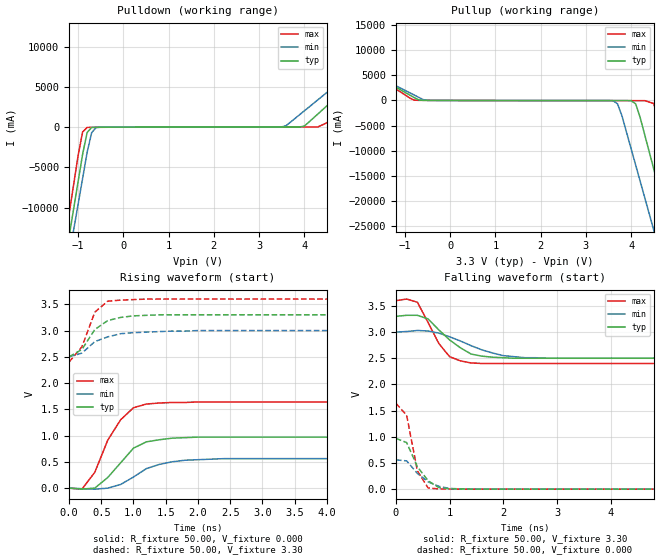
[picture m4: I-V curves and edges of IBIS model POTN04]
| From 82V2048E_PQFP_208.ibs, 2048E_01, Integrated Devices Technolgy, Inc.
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|   Model POTN04
[Model]   POTN04
Model_type   Output
Polarity   Non-Inverting
C_comp   3.50pF   4.00pF   3.50pF
[Temperature Range]   25.00   85.00   -40.00
[Voltage Range]   3.30V   3.00V   3.60V
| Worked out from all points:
|   slope of the pulldown table from 0 to 0.495 V, typ, clamps not added: 54.8 ohm
|   slope of the pullup table from 0 to 0.495 V, typ, clamps not added: 58.3 ohm
|   rising waveform, R_fixture 50.00, V_fixture 0.000: 20-80 % time 433ps typ, 533ps min, 401ps max; typ from -0.001 V to 0.97 V
|   rising waveform, R_fixture 50.00, V_fixture 3.30: 20-80 % time 331ps typ, 439ps min, 244ps max; typ from 2.5 V to 3.3 V
|   falling waveform, R_fixture 50.00, V_fixture 3.30: 20-80 % time 562ps typ, 775ps min, 404ps max; typ from 3.3 V to 2.5 V
|   falling waveform, R_fixture 50.00, V_fixture 0.000: 20-80 % time 325ps typ, 388ps min, 195ps max; typ from 0.97 V to 0 V
[Pulldown]
| voltage   I(typ)   I(min)   I(max)
-3.3V     -85.43A    -84.06A    -87.3A
-1.5V     -23.89A    -25.8A     -21.77A
-1V       -6.8A      -9.61A     -3.57A
-900mV    -3.38A     -6.38A     -600mA
-800mV    -670mA     -3.14A     -36.12mA
-700mV    -38.01mA   -680mA     -23.87mA
-600mV    -13.88mA   -49.26mA   -20.35mA
3.5V      16.11mA    21.26mA    24.2mA
4V        130mA      2.02A      24.28mA
4.3V      1.63A      3.39A      24.72mA
6.1V      10.82A     11.65A     9.85A
6.6V      13.37A     13.95A     12.77A
[Pullup]
| voltage   I(typ)   I(min)   I(max)
-3.3V     13.37A     12.57A     14.5A
-800mV    600mA      1.1A       64.98mA
-500mV    10.71mA    18.1mA     16.3mA
3.6V      -20.75mA   -52.54mA   -36.43mA
3.8V      -20.91mA   -3.15A     -36.66mA
4.1V      -680mA     -12.86A    -36.98mA
4.5V      -13.65A    -25.8A     -620mA
4.7V      -20.49A    -32.28A    -7.24A
4.9V      -27.33A    -38.75A    -14.52A
5.1V      -34.17A    -45.23A    -21.81A
5.3V      -41A       -51.7A     -29.09A
6.6V      -85.45A    -93.78A    -76.41A
[Ramp]
| variable   typ   min   max
dV/dt_r   0.58/0.47n   0.34/0.64n   0.98/0.34n
dV/dt_f   0.48/0.55n   0.30/0.72n   0.72/0.41n
R_load = 50.00
[Rising Waveform]
R_fixture = 50.00
V_fixture = 0.000
V_fixture_min = 0.000
V_fixture_max = 0.000
| time   V(typ)   V(min)   V(max)
0s        -1.1mV     -340uV     -2.04mV
200ps     -19.64mV   -13.03mV   -20.81mV
400ps     -930uV     -21.4mV    300mV
600ps     200mV      -1.92mV    910mV
800ps     480mV      67.78mV    1.3V
1ns       760mV      210mV      1.53V
1.2ns     880mV      370mV      1.6V
1.6ns     950mV      500mV      1.63V
2.4ns     970mV      560mV      1.64V
10ns      970mV      560mV      1.64V
[Rising Waveform]
R_fixture = 50.00
V_fixture = 3.30
V_fixture_min = 3.00
V_fixture_max = 3.60
| time   V(typ)   V(min)   V(max)
0s        2.5V       2.5V       2.4V
200ps     2.64V      2.57V      2.69V
400ps     3.02V      2.79V      3.35V
600ps     3.19V      2.88V      3.56V
800ps     3.25V      2.94V      3.58V
1ns       3.28V      2.96V      3.59V
1.2ns     3.29V      2.97V      3.6V
1.4ns     3.3V       2.98V      3.6V
2ns       3.3V       3V         3.6V
10ns      3.3V       3V         3.6V
[Falling Waveform]
R_fixture = 50.00
V_fixture = 3.30
V_fixture_min = 3.00
V_fixture_max = 3.60
| time   V(typ)   V(min)   V(max)
0s        3.3V       3V         3.6V
200ps     3.32V      3.01V      3.63V
400ps     3.32V      3.03V      3.57V
600ps     3.25V      3.02V      3.18V
800ps     3.04V      2.98V      2.78V
1ns       2.85V      2.91V      2.53V
1.4ns     2.58V      2.74V      2.41V
2ns       2.51V      2.55V      2.4V
2.4ns     2.5V       2.51V      2.4V
10ns      2.5V       2.5V       2.4V
[Falling Waveform]
R_fixture = 50.00
V_fixture = 0.000
V_fixture_min = 0.000
V_fixture_max = 0.000
| time   V(typ)   V(min)   V(max)
0s        970mV      560mV      1.64V
200ps     890mV      540mV      1.41V
400ps     430mV      300mV      350mV
600ps     160mV      140mV      21.96mV
800ps     29.25mV    54.03mV    4.56mV
1ns       6.83mV     12.93mV    2.15mV
1.2ns     3.23mV     6.4mV      860uV
2.4ns     160uV      350uV      93.03uV
10ns      220nV      3.02uV     1.1uV
